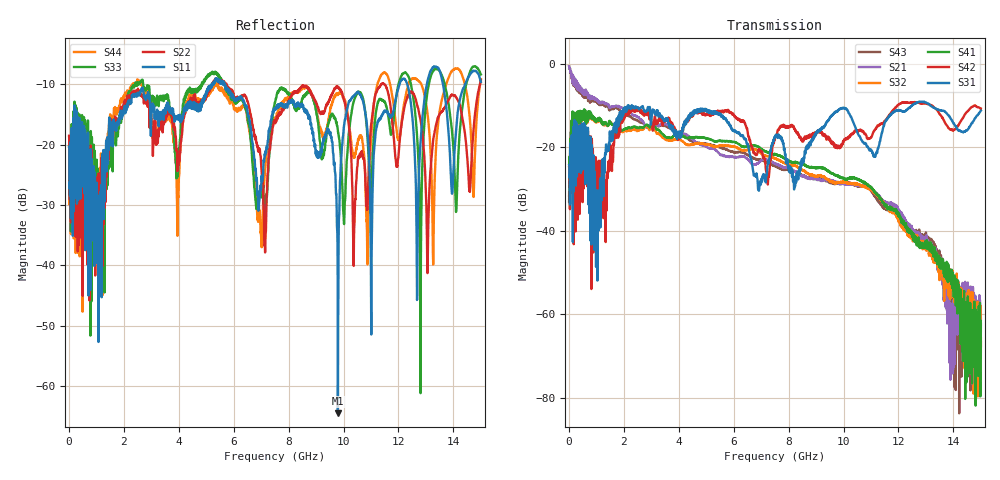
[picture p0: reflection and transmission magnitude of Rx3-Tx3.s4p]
! FILE: N:\QM 2007\Prüfprotokolle\Highspeed\Konfektionierte Ltg\L45593-D106\D30\8216\0002  kpl\IL  mit Chris Boards\Rx3-Tx3.s4p
# MHz S DB R 50.00
! FREQ  S11  S12  S13  S14
!  S21  S22  S23  S24
!  S31  S32  S33  S34
!  S41  S42  S43  S44
!  DB  ANG  DB  ANG  DB  ANG  DB  ANG
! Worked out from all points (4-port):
!   2999 points, 10 MHz to 15 GHz, reference 50 ohm
!   strongest paths, dB at 10 MHz, 3.755 GHz, 7.505 GHz, 11.26 GHz, 15 GHz:
!     S31: -24.2, -16.0, -17.5, -20.3, -11.2
!     S42: -24.8, -14.4, -18.0, -14.9, -10.8
!     S41: -33.0, -17.6, -21.6, -31.6, -62.3
!     S32: -31.6, -18.3, -22.6, -31.7, -65.8
!     S21: -0.6, -15.2, -23.8, -31.4, -61.1
!     S43: -0.6, -15.8, -24.4, -32.6, -67.6
!   lowest |S11| = -64.5 dB at 9.795 GHz (marker M1), VSWR 1.00, Z = 50.1 + j0.0222 ohm
!   |S11| at or under -10 dB: start of sweep to 5.212 GHz; 5.666 GHz to 12.04 GHz (6.374 GHz wide, 72 % of centre); 13.62 GHz to 14.43 GHz (804.6 MHz wide, 5.74 % of centre)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
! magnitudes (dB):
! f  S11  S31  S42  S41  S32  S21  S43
! 10 MHz  -20.4  -24.2  -24.8  -33.0  -31.6  -0.6  -0.6
! 5.375 GHz  -9.3  -11.9  -11.7  -18.5  -19.8  -20.8  -19.7
! 6.995 GHz  -27.5  -28.6  -21.1  -20.4  -21.5  -23.2  -23.0
! 8.13 GHz  -12.9  -26.5  -14.9  -23.6  -24.3  -25.3  -25.4
! 9.795 GHz  -64.5  -11.3  -19.8  -26.8  -28.4  -28.3  -28.6
! 13.06 GHz  -9.4  -9.5  -9.6  -44.3  -43.6  -42.9  -41.5
! 15 GHz  -9.6  -11.2  -10.8  -62.3  -65.8  -61.1  -67.6
